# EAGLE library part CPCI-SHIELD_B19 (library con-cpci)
Compact PCI - Abschirmblech unten B 19 / Lower Shield Type B 19 Source: www.erni.com
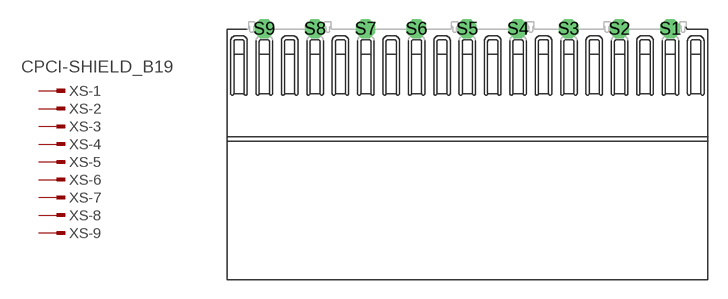
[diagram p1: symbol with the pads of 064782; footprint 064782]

Designator prefix XS; gates -1=PINV -2=PIN -3=PIN -4=PIN -5=PIN -6=PIN -7=PIN -8=PIN -9=PIN

## CPCI-SHIELD_B19 (OC_FARNELL: unknown; OC_NEWARK: unknown)  [064782]
S1  -1:1  in
S2  -2:1  in
S3  -3:1  in
S4  -4:1  in
S5  -5:1  in
S6  -6:1  in
S7  -7:1  in
S8  -8:1  in
S9  -9:1  in

## Footprint 064782 (pad centres in mm)
ERmet Abschirmblech unten B 19 / ERmet Lower Shield Type B 19 Source: http://www.erni.com/DB/PDF-Drawing/ERmet/064782.pdf
drill 1 octagon: S1 16,0; S2 12,0; S3 8,0; S4 4,0; S5 0,0; S6 -4,0; S7 -8,0; S8 -12,0; S9 -16,0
